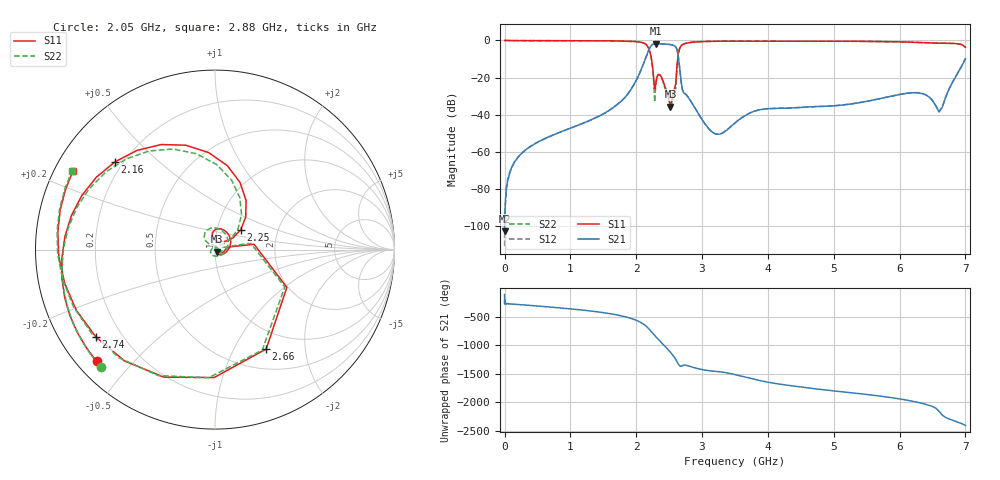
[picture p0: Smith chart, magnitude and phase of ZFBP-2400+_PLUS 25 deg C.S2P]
! Mini-Circuits
! S2P DATA File Format
! Type: BAND PASS FILTER
! Model: ZFBP-2400+
! All S Parameters are in dB deg format
! TEST CONDITIONS: INPUT POWER = 0 dBm @ Temperature = + 25 deg C
! 401 Frequency points
# MHz S DB R 50
!FREQMAG(S11)PHS(S11)MAG(S21)PHS(S21)MAG(S12)PHS(S12)MAG(S22)PHS(S22)
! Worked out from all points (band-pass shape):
!   401 points, 500 kHz to 7 GHz, reference 50 ohm
!   highest |S21| = -1.76 dB at 2.3 GHz (marker M1); lowest = -102.8 dB at 2 MHz (marker M2)
!   |S21| within 3 dB of the highest: 2.195 GHz to 2.617 GHz (421.2 MHz wide, 17.5 % of centre)
!   lowest |S11| = -35.6 dB at 2.52 GHz (marker M3), VSWR 1.03, Z = 51.1 - j1.26 ohm
!   |S11| at or under -10 dB: 2.231 GHz to 2.63 GHz (399.2 MHz wide, 16.4 % of centre)
!   |S22| runs from -36.6 to 0.0 dB; largest |S21 - S12| = 0.0012
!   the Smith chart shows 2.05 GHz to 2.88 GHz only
!   S11 on the Smith chart (normalised r, x): 2.05 GHz: 0.06, -0.40; 2.16 GHz: 0.17, +0.37; 2.25 GHz: 1.30, +0.30; 2.66 GHz: 0.75, -1.35; 2.74 GHz: 0.11, -0.32; 2.88 GHz: 0.05, +0.26
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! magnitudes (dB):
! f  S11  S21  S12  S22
! 500 kHz  0.0  -94.4  -110.9  0.0
! 2 MHz  0.0  -102.8  -97.2  0.0
! 290 MHz  -0.1  -59.9  -59.9  -0.1
! 1.17 GHz  -0.1  -44.9  -44.9  -0.1
! 1.77 GHz  -0.3  -32.8  -32.8  -0.3
! 2.05 GHz  -0.8  -17.8  -17.8  -0.8
! 2.16 GHz  -2.6  -7.8  -7.8  -2.5
! 2.25 GHz  -14.8  -2.1  -2.1  -15.2
! 2.27 GHz  -22.7  -1.8  -1.9  -25.4
! 2.3 GHz  -22.5  -1.8  -1.8  -23.0
! 2.34 GHz  -18.4  -1.8  -1.8  -18.3
! 2.52 GHz  -35.6  -2.2  -2.2  -35.3
! 2.56 GHz  -28.1  -2.5  -2.5  -29.9
! 2.66 GHz  -4.1  -14.9  -14.9  -4.2
! 2.74 GHz  -1.7  -28.7  -28.7  -1.6
! 2.88 GHz  -0.9  -35.7  -35.7  -0.8
! 3.2 GHz  -0.4  -50.3  -50.3  -0.4
! 3.52 GHz  -0.3  -43.9  -43.8  -0.3
! 4.7 GHz  -0.3  -35.7  -35.7  -0.4
! 5.85 GHz  -0.6  -30.2  -30.2  -0.7
! 6.6 GHz  -1.5  -38.5  -38.5  -1.4
! 7 GHz  -3.6  -9.9  -9.8  -3.6
